| IBIS file 70t3539z.ibs created by s2ibis2 version 1.1
| North Carolina State University Electronics Research Laboratory  1995
[IBIS ver]   2.1
[File name]   70t3539m.ibs
[File Rev]   4.0
|1.0 : Original Version - Wei-Ling Chang
|2.0 : Corrected Ramp rates and package RLC values - Wei-Ling Chang
|3.0 : Replaced I/O and Input models with ADC models - Sunil Kashyap
|4.0 : Corrected device identifier info.  Updated Package RLC. - Trevor Hiatt
[Date]   01/20/04
[Source]   Integrated Device Technology, Inc.
[Notes]   1. Temperatures: typ=25C, min=70C, max=0C 2. Cmos125_2.5v
   process. 3. Ramp rates based on 50 ohm load.
[Copyright]   Copyright 2003, Integrated Device Technology, Inc. Integrated
   Device Technology, Inc. ("IDT") hereby grants the user of this
   IBIS model a non-exclusive, nontransferable license to use
   this IBIS model under the following terms. The user is granted
   this license only to use the IBIS model and is not granted
   rights to sell, copy (except as needed to run the IBIS model),
   rent, lease or sub-license the IBIS model in whole or in part,
   or in modified form to anyone. The User may modify the IBIS
   model to suit its specific applications, but rights to
   derivative works and such modifications shall belong to IDT.
   This IBIS model is provided on an AS IS" basis and IDT makes
   absolutely no warranty with respect to the information
   contained herein. IDT DISCLAIMS AND CUSTOMER WAIVES ALL
   WARRANTIES, EXPRESS AND IMPLIED, INCLUDING WARRANTIES OF
   MERCHANTABILITY AND FITNESS FOR A PARTICULAR PURPOSE. THE
   ENTIRE RISK AS TO QUALITY AND PERFORMANCE IS WITH THE USER
   ACCORDINGLY, IN NO EVENT SHALL IDT BE LIABLE FOR ANY DIRECT OR
   INDIRECT DAMAGES, WHETHER IN CONTRACT OR TORT, INCLUDING ANY
   LOST PROFITS OR OTHER INCIDENTAL, CONSEQUENTIAL, EXEMPLARY, OR
   PUNITIVE DAMAGES ARISING OUT OF THE USE OR APPLICATION OF THE
   IBIS model. Further, IDT reserves the right to make changes
   without notice to any product herein to improve reliability,
   function, or design. IDT does not convey any license under
   patent rights or any other intellectual property rights,
   including those of third parties. IDT is not obligated to
   provide maintenance or support for the licensed IBIS model.
|   Component 70t3539z
[Component]   70t3539z
[Manufacturer]   Integrated Device Technology
[Package]
|256-pin BGA
| variable   typ   min   max
R_pkg   0.19   0.16   0.22
L_pkg   4.95nH   3.66nH   6.17nH
C_pkg   1.57pF   1.38pF   1.75pF
| NOTE:
| The model_name inpad25, inpadzz25, inpadbs25, and iopad25 work for
| both 3.3v and 2.5v vddq.  When vddq is 3.3v, the model names are
| inpad33, inpadzz33, inpadbs33, and iopad33.  When vddq is 2.5v,
| the model names will be inpad25, inpadzz25, inpadbs25,and iopad25.
[Pin]  signal_name   model_name   R_pin   L_pin   C_pin
C2   io19l   iopad25
D2   io19r   iopad25
D3   io20l   iopad25
D1   io20r   iopad25
D5   vddql   POWER
E7   intl#   iopad25
E2   io21l   iopad25
E1   io21r   iopad25
E3   io22l   iopad25
F2   io22r   iopad25
D7   vddqr   POWER
E8   vss   GND
F1   io23l   iopad25
F3   io23r   iopad25
G2   io24l   iopad25
G1   io24r   iopad25
D6   vddql   POWER
F6   vss   GND
G3   io25l   iopad25
H2   io25r   iopad25
H1   io26l   iopad25
H3   io26r   iopad25
G4   vddqr   POWER
G5   vss   GND
E5   vdd   POWER
G6   vss   GND
E4   vddql   POWER
C3   vss   GND
J3   io27r   iopad25
J1   io27l   iopad25
J2   io28r   iopad25
K3   io28l   iopad25
H4   vddqr   POWER
H5   vss   GND
K1   io29r   iopad25
K2   io29l   iopad25
L3   io30r   iopad25
L1   io30l   iopad25
J4   vddql   POWER
J5   zzr   inpadzz25
L2   io31r   iopad25
M3   io31l   iopad25
M1   io32r   iopad25
M2   io32l   iopad25
L4   vddqr   POWER
L6   vss   GND
N3   io33r   iopad25
N1   io33l   iopad25
N2   io34r   iopad25
P2   io34l   iopad25
P1   io35r   iopad25
R1   io35l   iopad25
M7   intl#   iopad25
R4   a18r   inpad25
T4   a17r   inpad25
P4   a16r   inpad25
R5   a15r   inpad25
T5   a14r   inpad25
P5   a13r   inpad25
R6   a12r   inpad25
T6   a11r   inpad25
P6   a10r   inpad25
R7   a9r   inpad25
T7   a8r   inpad25
P7   a7r   inpad25
R8   be3r#   inpad25
T8   be2r#   inpad25
P8   be1r#   inpad25
P9   be0r#   inpad25
T9   ce1r   inpad25
R9   ce0r#   inpad25
N13   vdd   POWER
M12   vdd   POWER
M9   vss   GND
M10   vss   GND
P10   clkr   inpad25
T10   oer#   inpad25
R10   rwr#   inpad25
P11   adsr#   inpad25
T11   cntenr#  inpad25
R11   repeatr# inpad25
P12   a6r   inpad25
T12   a5r   inpad25
R12   a4r   inpad25
P13   a3r   inpad25
T13   a2r   inpad25
R13   a1r   inpad25
T14   a0r   inpad25
M11   vdd   POWER
M8   vss   GND
M6   vdd   POWER
P14   io0l   iopad25
P15   io0r   iopad25
N12   vddql   POWER
L11   vss   GND
P16   io1l   iopad25
N15   io1r   iopad25
N14   io2l   iopad25
N16   io2r   iopad25
N10   vddqr   POWER
L10   vss   GND
M15   io3l   iopad25
M14   io3r   iopad25
M16   io4l   iopad25
L15   io4r   iopad25
N11   vddql   POWER
L9   vss   GND
L14   io5l   iopad25
L16   io5r   iopad25
K15   io6l   iopad25
K14   io6r   iopad25
K13   vddqr   POWER
K12   vss   GND
K16   io7l   iopad25
J15   io7r   iopad25
J16   io8l   iopad25
J14   io8r   iopad25
M13   vddql   POWER
K9   vss   GND
K10   vss   GND
K11   vss   GND
L12   vdd   POWER
M5   vdd   POWER
N9   vddqr   POWER
L8   vss   GND
H14   io9r   iopad25
H15   io9l   iopad25
H16   io10r   iopad25
G14   io10l   iopad25
L13   vddql   POWER
L7   colr#   iopad25
G16   io11r   iopad25
G15   io11l   iopad25
F14   io12r   iopad25
F16   io12l   iopad25
J13   vddqr   POWER
J12   zzl   inpadzz25
F15   io13r   iopad25
E14   io13l   iopad25
E16   io14r   iopad25
E15   io14l   iopad25
H13   vddql   POWER
H12   vss   GND
D14   io15r   iopad25
D15   io15l   iopad25
D16   io16r   iopad25
C16   io16l   iopad25
G12   vss   GND
F13   vddqr   POWER
C15   io17r   iopad25
B15   io17l   iopad25
L5   vdd   POWER
F11   vss   GND
F5   vdd   POWER
D13   vdd   POWER
A14   a0l   inpad25
B13   a1l   inpad25
A13   a2l   inpad25
C13   a3l   inpad25
B12   a4l   inpad25
A12   a5l   inpad25
C12   a6l   inpad25
B11   repeatl# inpad25
A11   cntenl#  inpad25
C11   adsl#   inpad25
B10   rwl#   inpad25
A10   oel#   inpad25
C10   clkl   inpad25
E9   vss   GND
E10   vss   GND
B14   vdd   POWER
E6   vdd   POWER
B9   ce0l   inpad25
A9   ce1l   inpad25
C9   be0l#   inpad25
C8   be1l#   inpad25
A8   be2l#   inpad25
B8   be3l#   inpad25
C7   a7l   inpad25
A7   a8l   inpad25
B7   a9l   inpad25
C6   a10l   inpad25
A6   a11l   inpad25
B6   a12l   inpad25
C5   a13l   inpad25
A5   a14l   inpad25
B5   a15l   inpad25
C4   a16l   inpad25
A4   a17l   inpad25
B4   a18l   inpad25
F9   vss   GND
E11   vdd   POWER
F10   vss   GND
B1   io18l   iopad25
C1   io18r   iopad25
D12   vddqr   POWER
F8   vss   GND
R14   optr   inpad25
C14   optl   inpad25
D11   vddqr   POWER
E13   vddqr   POWER
N5   vddqr   POWER
N6   vddqr   POWER
D8   vddqr   POWER
M4   vddqr   POWER
G13   vddql   POWER
F4   vddql   POWER
D9   vddql   POWER
D10   vddql   POWER
K4   vddql   POWER
N7   vddql   POWER
N8   vddql   POWER
E12   vdd   POWER
F12   vdd   POWER
F7   coll#   iopad25
G7   vss   GND
G8   vss   GND
G9   vss   GND
G10   vss   GND
G11   vss   GND
H6   vss   GND
H7   vss   GND
H8   vss   GND
H9   vss   GND
H10   vss   GND
H11   vss   GND
J6   vss   GND
J7   vss   GND
J8   vss   GND
J9   vss   GND
J10   vss   GND
J11   vss   GND
K5   vss   GND
K6   vss   GND
K7   vss   GND
K8   vss   GND
N4   plftr#   inpad25
D4   plftl#   inpad25
P3   tms   inpadbs25
T2   tck   inpadbs25
R3   trst#   inpadbs25
A2   tdi   inpadbs25
B3   tdo   iopad25
| NDAIN NDAIN   dummy_model
| OC   OC   dummy_model
| PUD   PUD   dummy_model|
[Pin Mapping]  pulldown_ref   pullup_ref   gnd_clamp_ref   power_clamp_ref
C2 EXTGND   EXTVDDQ   EXTGND   EXTVDD
D2 EXTGND   EXTVDDQ   EXTGND   EXTVDD
D3 EXTGND   EXTVDDQ   EXTGND   EXTVDD
D1 EXTGND   EXTVDDQ   EXTGND   EXTVDD
D5 NC  EXTVDDQ
E7 EXTGND   EXTVDDQ   EXTGND   EXTVDD
E2 EXTGND   EXTVDDQ   EXTGND   EXTVDD
E1 EXTGND   EXTVDDQ   EXTGND   EXTVDD
E3 EXTGND   EXTVDDQ   EXTGND   EXTVDD
F2 EXTGND   EXTVDDQ   EXTGND   EXTVDD
D7 NC  EXTVDDQ
E8 EXTGND   NC
F1 EXTGND   EXTVDDQ   EXTGND   EXTVDD
F3 EXTGND   EXTVDDQ   EXTGND   EXTVDD
G2 EXTGND   EXTVDDQ   EXTGND   EXTVDD
G1 EXTGND   EXTVDDQ   EXTGND   EXTVDD
D6 NC  EXTVDDQ
F6 EXTGND   NC
G3 EXTGND   EXTVDDQ   EXTGND   EXTVDD
H2 EXTGND   EXTVDDQ   EXTGND   EXTVDD
H1 EXTGND   EXTVDDQ   EXTGND   EXTVDD
H3 EXTGND   EXTVDDQ   EXTGND   EXTVDD
G4 NC  EXTVDDQ
G5 EXTGND   NC
E5 NC  EXTVDD
G6 EXTGND   NC
E4 NC  EXTVDDQ
C3 EXTGND   NC
J3 EXTGND   EXTVDDQ   EXTGND   EXTVDD
J1 EXTGND   EXTVDDQ   EXTGND   EXTVDD
J2 EXTGND   EXTVDDQ   EXTGND   EXTVDD
K3 EXTGND   EXTVDDQ   EXTGND   EXTVDD
H4 NC  EXTVDDQ
H5 EXTGND   NC
K1 EXTGND   EXTVDDQ   EXTGND   EXTVDD
K2 EXTGND   EXTVDDQ   EXTGND   EXTVDD
L3 EXTGND   EXTVDDQ   EXTGND   EXTVDD
L1 EXTGND   EXTVDDQ   EXTGND   EXTVDD
J4 NC  EXTVDDQ
J5 EXTGND   EXTVDDQ   EXTGND   EXTVDD
L2 EXTGND   EXTVDDQ   EXTGND   EXTVDD
M3 EXTGND   EXTVDDQ   EXTGND   EXTVDD
M1 EXTGND   EXTVDDQ   EXTGND   EXTVDD
M2 EXTGND   EXTVDDQ   EXTGND   EXTVDD
L4 NC  EXTVDDQ
L6 EXTGND   NC
N3 EXTGND   EXTVDDQ   EXTGND   EXTVDD
N1 EXTGND   EXTVDDQ   EXTGND   EXTVDD
N2 EXTGND   EXTVDDQ   EXTGND   EXTVDD
P2 EXTGND   EXTVDDQ   EXTGND   EXTVDD
P1 EXTGND   EXTVDDQ   EXTGND   EXTVDD
R1 EXTGND   EXTVDDQ   EXTGND   EXTVDD
M7 EXTGND   EXTVDDQ   EXTGND   EXTVDD
R4 EXTGND   EXTVDDQ   EXTGND   EXTVDD
T4 EXTGND   EXTVDDQ   EXTGND   EXTVDD
P4 EXTGND   EXTVDDQ   EXTGND   EXTVDD
R5 EXTGND   EXTVDDQ   EXTGND   EXTVDD
T5 EXTGND   EXTVDDQ   EXTGND   EXTVDD
P5 EXTGND   EXTVDDQ   EXTGND   EXTVDD
R6 EXTGND   EXTVDDQ   EXTGND   EXTVDD
T6 EXTGND   EXTVDDQ   EXTGND   EXTVDD
P6 EXTGND   EXTVDDQ   EXTGND   EXTVDD
R7 EXTGND   EXTVDDQ   EXTGND   EXTVDD
T7 EXTGND   EXTVDDQ   EXTGND   EXTVDD
P7 EXTGND   EXTVDDQ   EXTGND   EXTVDD
R8 EXTGND   EXTVDDQ   EXTGND   EXTVDD
T8 EXTGND   EXTVDDQ   EXTGND   EXTVDD
P8 EXTGND   EXTVDDQ   EXTGND   EXTVDD
P9 EXTGND   EXTVDDQ   EXTGND   EXTVDD
T9 EXTGND   EXTVDDQ   EXTGND   EXTVDD
R9 EXTGND   EXTVDDQ   EXTGND   EXTVDD
N13   NC  EXTVDD
M12   NC  EXTVDD
M9 EXTGND   NC
M10   EXTGND   NC
P10   EXTGND   EXTVDDQ   EXTGND   EXTVDD
T10   EXTGND   EXTVDDQ   EXTGND   EXTVDD
R10   EXTGND   EXTVDDQ   EXTGND   EXTVDD
P11   EXTGND   EXTVDDQ   EXTGND   EXTVDD
T11   EXTGND   EXTVDDQ   EXTGND   EXTVDD
R11   EXTGND   EXTVDDQ   EXTGND   EXTVDD
P12   EXTGND   EXTVDDQ   EXTGND   EXTVDD
T12   EXTGND   EXTVDDQ   EXTGND   EXTVDD
R12   EXTGND   EXTVDDQ   EXTGND   EXTVDD
P13   EXTGND   EXTVDDQ   EXTGND   EXTVDD
T13   EXTGND   EXTVDDQ   EXTGND   EXTVDD
R13   EXTGND   EXTVDDQ   EXTGND   EXTVDD
T14   EXTGND   EXTVDDQ   EXTGND   EXTVDD
M11   NC  EXTVDD
M8 EXTGND   NC
M6 NC  EXTVDD
P14   EXTGND   EXTVDDQ   EXTGND   EXTVDD
P15   EXTGND   EXTVDDQ   EXTGND   EXTVDD
N12   NC  EXTVDDQ
L11   EXTGND   NC
P16   EXTGND   EXTVDDQ   EXTGND   EXTVDD
N15   EXTGND   EXTVDDQ   EXTGND   EXTVDD
N14   EXTGND   EXTVDDQ   EXTGND   EXTVDD
N16   EXTGND   EXTVDDQ   EXTGND   EXTVDD
N10   NC  EXTVDDQ
L10   EXTGND   NC
M15   EXTGND   EXTVDDQ   EXTGND   EXTVDD
M14   EXTGND   EXTVDDQ   EXTGND   EXTVDD
M16   EXTGND   EXTVDDQ   EXTGND   EXTVDD
L15   EXTGND   EXTVDDQ   EXTGND   EXTVDD
N11   NC  EXTVDDQ
L9 EXTGND   NC
L14   EXTGND   EXTVDDQ   EXTGND   EXTVDD
L16   EXTGND   EXTVDDQ   EXTGND   EXTVDD
K15   EXTGND   EXTVDDQ   EXTGND   EXTVDD
K14   EXTGND   EXTVDDQ   EXTGND   EXTVDD
K13   NC  EXTVDDQ
K12   EXTGND   NC
K16   EXTGND   EXTVDDQ   EXTGND   EXTVDD
J15   EXTGND   EXTVDDQ   EXTGND   EXTVDD
J16   EXTGND   EXTVDDQ   EXTGND   EXTVDD
J14   EXTGND   EXTVDDQ   EXTGND   EXTVDD
M13   NC  EXTVDDQ
K9 EXTGND   NC
K10   EXTGND   NC
K11   EXTGND   NC
L12   NC  EXTVDD
M5 NC  EXTVDD
N9 NC  EXTVDDQ
L8 EXTGND   NC
H14   EXTGND   EXTVDDQ   EXTGND   EXTVDD
H15   EXTGND   EXTVDDQ   EXTGND   EXTVDD
H16   EXTGND   EXTVDDQ   EXTGND   EXTVDD
G14   EXTGND   EXTVDDQ   EXTGND   EXTVDD
L13   NC  EXTVDDQ
L7   EXTGND   EXTVDDQ   EXTGND   EXTVDD
G16   EXTGND   EXTVDDQ   EXTGND   EXTVDD
G15   EXTGND   EXTVDDQ   EXTGND   EXTVDD
F14   EXTGND   EXTVDDQ   EXTGND   EXTVDD
F16   EXTGND   EXTVDDQ   EXTGND   EXTVDD
J13   NC  EXTVDDQ
J12   EXTGND   EXTVDDQ   EXTGND   EXTVDD
F15   EXTGND   EXTVDDQ   EXTGND   EXTVDD
E14   EXTGND   EXTVDDQ   EXTGND   EXTVDD
E16   EXTGND   EXTVDDQ   EXTGND   EXTVDD
E15   EXTGND   EXTVDDQ   EXTGND   EXTVDD
H13   NC  EXTVDDQ
H12   EXTGND   NC
D14   EXTGND   EXTVDDQ   EXTGND   EXTVDD
D15   EXTGND   EXTVDDQ   EXTGND   EXTVDD
D16   EXTGND   EXTVDDQ   EXTGND   EXTVDD
C16   EXTGND   EXTVDDQ   EXTGND   EXTVDD
G12   EXTGND   NC
F13   NC  EXTVDDQ
C15   EXTGND   EXTVDDQ   EXTGND   EXTVDD
B15   EXTGND   EXTVDDQ   EXTGND   EXTVDD
L5 NC  EXTVDD
F11   EXTGND   NC
F5 NC  EXTVDD
D13   NC  EXTVDD
A14   EXTGND   EXTVDDQ   EXTGND   EXTVDD
B13   EXTGND   EXTVDDQ   EXTGND   EXTVDD
A13   EXTGND   EXTVDDQ   EXTGND   EXTVDD
C13   EXTGND   EXTVDDQ   EXTGND   EXTVDD
B12   EXTGND   EXTVDDQ   EXTGND   EXTVDD
A12   EXTGND   EXTVDDQ   EXTGND   EXTVDD
C12   EXTGND   EXTVDDQ   EXTGND   EXTVDD
B11   EXTGND   EXTVDDQ   EXTGND   EXTVDD
A11   EXTGND   EXTVDDQ   EXTGND   EXTVDD
C11   EXTGND   EXTVDDQ   EXTGND   EXTVDD
B10   EXTGND   EXTVDDQ   EXTGND   EXTVDD
A10   EXTGND   EXTVDDQ   EXTGND   EXTVDD
C10   EXTGND   EXTVDDQ   EXTGND   EXTVDD
E9 EXTGND   NC
E10   EXTGND   NC
B14   NC  EXTVDD
E6 NC  EXTVDD
B9 EXTGND   EXTVDDQ   EXTGND   EXTVDD
A9 EXTGND   EXTVDDQ   EXTGND   EXTVDD
C9 EXTGND   EXTVDDQ   EXTGND   EXTVDD
C8 EXTGND   EXTVDDQ   EXTGND   EXTVDD
A8 EXTGND   EXTVDDQ   EXTGND   EXTVDD
B8 EXTGND   EXTVDDQ   EXTGND   EXTVDD
C7 EXTGND   EXTVDDQ   EXTGND   EXTVDD
A7 EXTGND   EXTVDDQ   EXTGND   EXTVDD
B7 EXTGND   EXTVDDQ   EXTGND   EXTVDD
C6 EXTGND   EXTVDDQ   EXTGND   EXTVDD
A6 EXTGND   EXTVDDQ   EXTGND   EXTVDD
B6 EXTGND   EXTVDDQ   EXTGND   EXTVDD
C5 EXTGND   EXTVDDQ   EXTGND   EXTVDD
A5 EXTGND   EXTVDDQ   EXTGND   EXTVDD
B5 EXTGND   EXTVDDQ   EXTGND   EXTVDD
C4 EXTGND   EXTVDDQ   EXTGND   EXTVDD
A4 EXTGND   EXTVDDQ   EXTGND   EXTVDD
B4 EXTGND   EXTVDDQ   EXTGND   EXTVDD
F9 EXTGND   NC
E11   NC  EXTVDD
F10   EXTGND   NC
B1 EXTGND   EXTVDDQ   EXTGND   EXTVDD
C1 EXTGND   EXTVDDQ   EXTGND   EXTVDD
D12   NC  EXTVDDQ
F8 EXTGND   NC
R14   EXTGND   EXTVDDQ   EXTGND   EXTVDD
C14   EXTGND   EXTVDDQ   EXTGND   EXTVDD
D11   NC  EXTVDDQ
E13   NC  EXTVDDQ
N5 NC  EXTVDDQ
N6 NC  EXTVDDQ
D8 NC  EXTVDDQ
M4 NC  EXTVDDQ
G13   NC  EXTVDDQ
F4 NC  EXTVDDQ
D9 NC  EXTVDDQ
D10   NC  EXTVDDQ
K4 NC  EXTVDDQ
N7 NC  EXTVDDQ
N8 NC  EXTVDDQ
E12   NC  EXTVDD
F12   NC  EXTVDD
F7 EXTGND   EXTVDDQ   EXTGND   EXTVDD
G7 EXTGND   NC
G8 EXTGND   NC
G9 EXTGND   NC
G10   EXTGND   NC
G11   EXTGND   NC
H6 EXTGND   NC
H7 EXTGND   NC
H8 EXTGND   NC
H9 EXTGND   NC
H10   EXTGND   NC
H11   EXTGND   NC
J6 EXTGND   NC
J7 EXTGND   NC
J8 EXTGND   NC
J9 EXTGND   NC
J10   EXTGND   NC
J11   EXTGND   NC
K5 EXTGND   NC
K6 EXTGND   NC
K7 EXTGND   NC
K8 EXTGND   NC
N4 EXTGND   EXTVDDQ   EXTGND   EXTVDD
D4 EXTGND   EXTVDDQ   EXTGND   EXTVDD
P3 EXTGND   EXTVDDQ   EXTGND   EXTVDD
T2 EXTGND   EXTVDDQ   EXTGND   EXTVDD
R3 EXTGND   EXTVDDQ   EXTGND   EXTVDD
A2 EXTGND   EXTVDDQ   EXTGND   EXTVDD
B3 EXTGND   EXTVDDQ   EXTGND   EXTVDD
| Models and submodels in the file (8): inpad25 (Input), inpad33 (Input), inpadzz25 (Input), inpadzz33 (Input), inpadbs25 (Input), inpadbs33 (Input), iopad25 (I/O), iopad33 (I/O)
